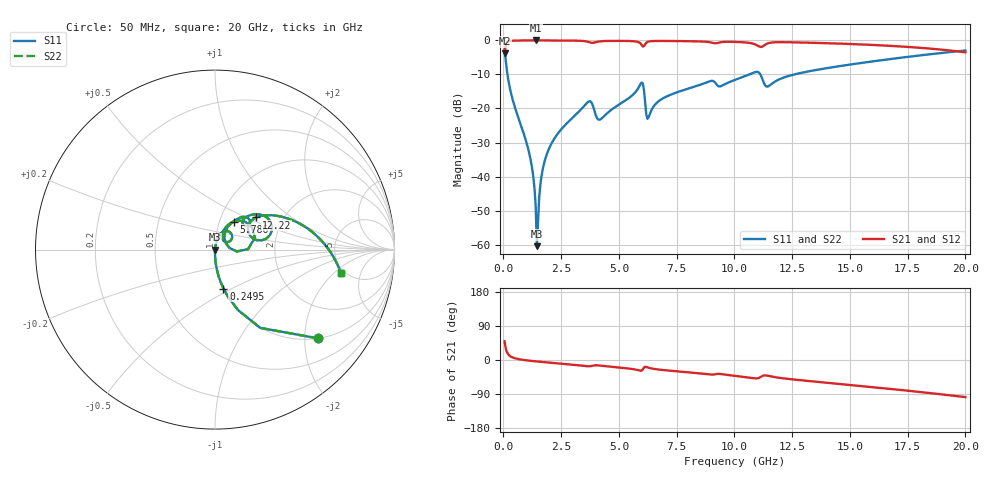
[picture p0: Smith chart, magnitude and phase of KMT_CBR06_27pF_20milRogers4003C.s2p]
! Data measured by Modelithics Inc. support@modelithics.com 813-866-6335
! KEMET CBR0603 27pF, Pad Width= 0.851mm, Pad Length= 0.64mm, Pad Gap= 0.62mm, 20mil Rogers 4003C substrate Data, January 2022
# hz S ma R 50
! 2 Port Network Data from SP1.SP block
! freq  magS11  angS11  magS21  angS21  magS12  angS12  magS22  angS22
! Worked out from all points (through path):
!   401 points, 50 MHz to 20 GHz, reference 50 ohm
!   highest |S21| = -0.01 dB at 1.397 GHz (marker M1); lowest = -3.7 dB at 50 MHz (marker M2)
!   group delay of S21, straight-line fit = 13.7 ps
!   lowest |S11| = -60.5 dB at 1.446 GHz (marker M3), VSWR 1.00, Z = 50.1 - j0.0713 ohm
!   |S11| at or under -10 dB: 174.4 MHz to 10.65 GHz (10.47 GHz wide, 194 % of centre); 11.13 GHz to 12.59 GHz (1.465 GHz wide, 12.4 % of centre)
!   |S22| runs from -60.5 to -2.4 dB; largest |S21 - S12| = 0
!   S11 on the Smith chart (normalised r, x): 50 MHz: 1.00, -2.33; 249.5 MHz: 1.00, -0.45; 5.786 GHz: 1.17, +0.38; 12.22 GHz: 1.46, +0.57; 20 GHz: 4.63, -2.43
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5e7  0.7596 -40.7  0.6498 49.3  0.6498 49.3  0.7596 -40.7
2.495e8  0.222 -77.7  0.9746 12.2  0.9746 12.2  0.222 -77.7
1.14725e9  0.0197 -90.2  0.9992 -1.9  0.9992 -1.9  0.0197 -90.2
1.396625e9  0.003602 -83.0  0.9993 -3.5  0.9993 -3.5  0.003602 -83.0
1.4465e9  0.0009474 -48.7  0.9993 -3.8  0.9993 -3.8  0.0009474 -48.7
1.54625e9  0.004869 77.3  0.9992 -4.4  0.9992 -4.4  0.004869 77.3
1.695875e9  0.01256 81.4  0.9991 -5.2  0.9991 -5.2  0.01256 81.4
1.995125e9  0.02677 81.3  0.9987 -6.9  0.9987 -6.9  0.02677 81.3
3.391625e9  0.0996 69.4  0.9848 -14.7  0.9848 -14.7  0.0996 69.4
3.74075e9  0.128 47.3  0.9369 -16.6  0.9369 -16.6  0.128 47.3
4.189625e9  0.06894 51.0  0.9696 -14.8  0.9696 -14.8  0.06894 51.0
5.785625e9  0.1871 56.3  0.9577 -26.1  0.9577 -26.1  0.1871 56.3
5.985125e9  0.2412 32.2  0.8578 -28.0  0.8578 -28.0  0.2412 32.2
6.284375e9  0.07425 41.5  0.9627 -20.5  0.9627 -20.5  0.07425 41.5
6.73325e9  0.1291 61.0  0.983 -25.3  0.983 -25.3  0.1291 61.0
1.0025e10  0.2629 45.4  0.9516 -41.8  0.9516 -41.8  0.2629 45.4
1.097262e10  0.3458 26.0  0.8501 -48.5  0.8501 -48.5  0.3458 26.0
1.127188e10  0.2386 12.7  0.8391 -40.8  0.8391 -40.8  0.2386 12.7
1.22195e10  0.2915 38.0  0.9416 -49.2  0.9416 -49.2  0.2915 38.0
1.336662e10  0.3592 32.3  0.9238 -56.3  0.9238 -56.3  0.3592 32.3
1.670825e10  0.5304 12.7  0.8343 -76.0  0.8343 -76.0  0.5304 12.7
2e10  0.7123 -10.4  0.6695 -97.9  0.6695 -97.9  0.7123 -10.4
